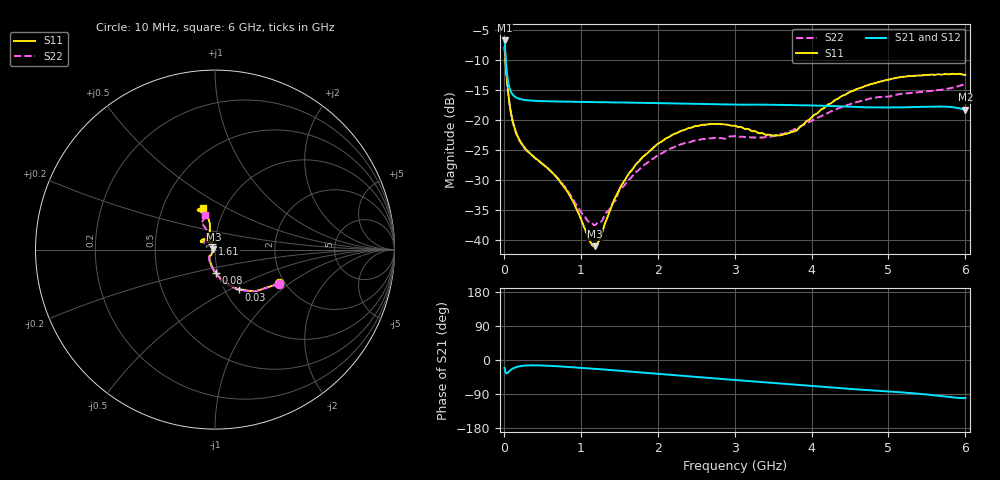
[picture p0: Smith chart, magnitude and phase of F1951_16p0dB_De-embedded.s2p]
! Integrated Device Technology
! Corporate Headquarters
! 6024 Silver Creek Valley Road
! San Jose, CA 95138  USA
! Phone:  1-408-284-8200
! Toll Free:  1-800-223-1366
! Webpage:  http://www.idt.com/
! Timing and RF Division
! 515 Groton Road, Suite 102
! Westford, MA 01886-6024
! Device:  F1951
! Description: 6-bit 0.5 dB Digital Step Attenuator
! Frequency:  100.0 -  4000.00 MHz
! Package:  4x4 mm Thin QFN Plastic Package: 24 pin
! Ports:  2 RF, 6 DC
!  Pin  1  = NC
!  Pin  2  = RF1  =  Port 1
!  Pin  3  = GND
!  Pin  4  = NC
!  Pin  5  = Serial Data Out (SDO)
!  Pin  6  = NC
!  Pin  7  = Reset Bar ( RSTb)
!  Pin  8  = Clock (CLK)
!  Pin  9  = Chip Select Bar (CSb)
!  Pin 10  = NC
!  Pin 11  = Serial Data In (SDI)
!  Pin 12  = NC
!  Pin 13  = NC
!  Pin 14  = VDD
!  Pin 15  = NC
!  Pin 16  = GND
!  Pin 17  = RF2  =  Port 2
!  Pin 18  = NC
!  Pin 19  = GND
!  Pin 20  = GND
!  Pin 21  = GND
!  Pin 22  = GND
!  Pin 23  = GND
!  Pin 24  = GND
! State:  32
! Atten State:  16.0 dB
! Voltage:  +3.30 Volts
! Current:  0.477 mA
! Data:  The device was measured on a F195X evaluation board which has
!  individual transmission lines to the RF pins.  Data was collected
!  de-embedded using a Automatic Fixture Removal [AFR] (Keysight Technologies).
!  The reference plane is the edge of the package pin.
! Misc:  Lot Code  1225BCA
!  Action Tracker AT0399
! Date Measured:  2018-09-13
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# GHz S dB R 50
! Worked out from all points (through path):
!   600 points, 10 MHz to 6 GHz, reference 50 ohm
!   highest |S21| = -6.69 dB at 10 MHz (marker M1); lowest = -18.2 dB at 6 GHz (marker M2)
!   group delay of S21, straight-line fit = 41.7 ps
!   lowest |S11| = -41.0 dB at 1.18 GHz (marker M3), VSWR 1.02, Z = 49.1 + j0.089 ohm
!   |S11| at or under -10 dB: 20.91 MHz to end of sweep
!   |S22| runs from -37.5 to -7.9 dB; largest |S21 - S12| = 0.00032
!   S11 on the Smith chart (normalised r, x): 10 MHz: 1.87, -0.84; 30 MHz: 1.17, -0.56; 80 MHz: 0.98, -0.26; 1.61 GHz: 0.97, +0.06; 6 GHz: 0.79, +0.39
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0.01  -7.87 -27.8  -6.69 -20.7  -6.69 -20.7  -7.89 -28.4
0.03  -11.69 -58.6  -10.58 -35.0  -10.58 -35.1  -11.77 -59.8
0.08  -17.75 -88.0  -14.83 -27.9  -14.84 -27.9  -17.88 -90.0
0.15  -21.70 -106.6  -16.13 -19.5  -16.12 -19.4  -21.81 -108.8
0.25  -24.22 -119.2  -16.56 -15.2  -16.56 -15.1  -24.35 -122.4
0.71  -29.84 -127.2  -16.86 -16.6  -16.86 -16.7  -29.81 -136.2
0.87  -32.83 -129.0  -16.91 -18.8  -16.91 -18.8  -32.51 -140.8
1.01  -36.72 -137.2  -16.95 -20.7  -16.95 -20.7  -35.41 -150.0
1.12  -40.18 -161.3  -16.96 -22.2  -16.96 -22.2  -36.93 -166.9
1.18  -40.97 174.2  -16.97 -23.2  -16.97 -23.2  -37.48 -179.9
1.27  -39.04 141.4  -16.98 -24.6  -16.98 -24.5  -36.84 161.3
1.43  -33.35 121.6  -17.01 -27.2  -17.01 -27.1  -33.58 140.4
1.61  -29.15 118.6  -17.04 -30.0  -17.04 -30.0  -30.14 131.6
2.01  -23.85 127.2  -17.13 -36.6  -17.13 -36.6  -25.72 133.8
2.49  -20.95 140.5  -17.25 -44.5  -17.25 -44.5  -23.37 142.1
3.01  -20.92 150.8  -17.37 -52.8  -17.37 -52.8  -22.63 146.1
3.59  -22.51 130.2  -17.42 -62.0  -17.42 -62.0  -22.33 128.1
3.79  -21.80 115.5  -17.49 -65.3  -17.49 -65.2  -21.41 121.3
4.01  -19.39 105.7  -17.51 -68.8  -17.52 -68.8  -20.05 115.9
4.49  -15.31 101.9  -17.73 -76.1  -17.73 -76.1  -17.35 114.4
5.01  -13.20 109.7  -17.85 -83.0  -17.85 -83.0  -16.03 117.1
6  -12.41 105.9  -18.21 -100.6  -18.21 -100.6  -13.92 105.7
